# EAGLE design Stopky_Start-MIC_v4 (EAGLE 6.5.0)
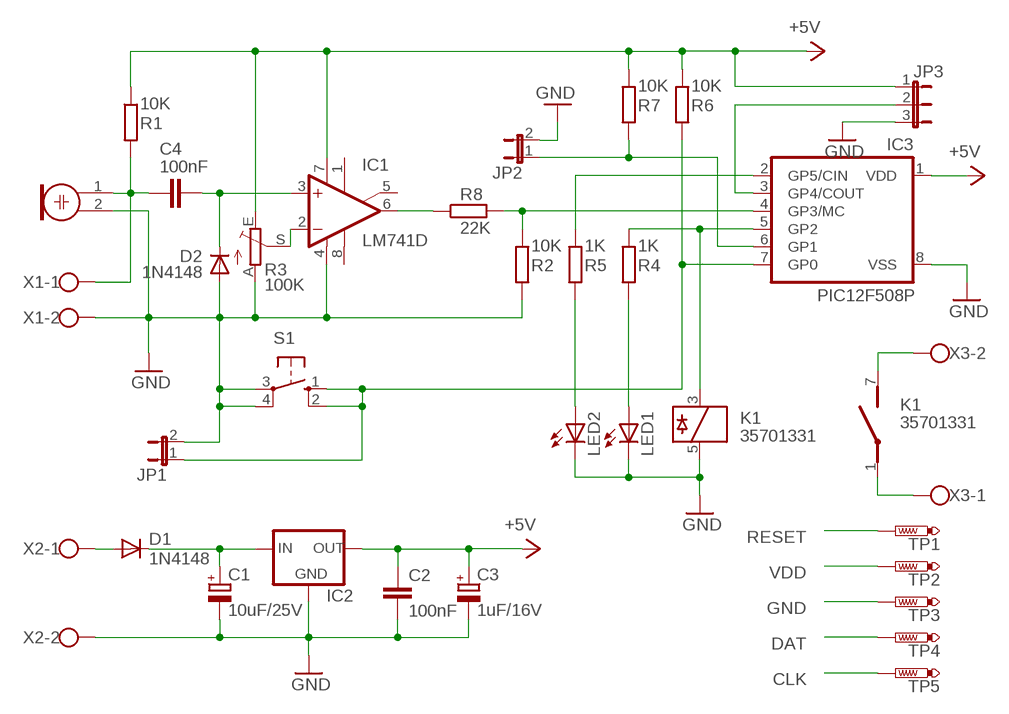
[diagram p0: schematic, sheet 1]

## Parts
C1  10uF/25V  CPOL-EUSMCD  [SMC_D]
C2  100nF  C-EUC1206  [C1206]
C3  1uF/16V  CPOL-EUSMCA  [SMC_A]
C4  100nF  C-EUC1206  [C1206]
D1  1N4148  PMLL4150  [SOD80C]
D2  1N4148  PMLL4150  [SOD80C]
IC1  LM741D  [SO08]
IC2  78LXX-SOT89  [SOT89]
IC3  PIC12F508P  PIC12C508P  [DIL8]
JP1  JP1E  [JP1]
JP2  JP1E  [JP1]
JP3  JP2E  [JP2]
K1  35701331  [REED]
LED1  LED3MM  [LED3MM]
LED2  LED3MM  [LED3MM]
M1  ELECTRET_MIC  ELECTRET_MICROPHON-F6050AP  [F6050AP]
R1  10K  R-EU_R1206  [R1206]
R2  10K  R-EU_R1206  [R1206]
R3  100K  TRIM_EU-CA6V  [CA6V]
R4  1K  R-EU_R1206  [R1206]
R5  1K  R-EU_R1206  [R1206]
R6  10K  R-EU_R1206  [R1206]
R7  10K  R-EU_R1206  [R1206]
R8  22K  R-EU_R1206  [R1206]
S1  10-XX  [B3F-10XX]
TP1  PTR1TP15R  [TP15R]
TP2  PTR1TP15R  [TP15R]
TP3  PTR1TP15R  [TP15R]
TP4  PTR1TP15R  [TP15R]
TP5  PTR1TP15R  [TP15R]
X1  AK550/2  [AK550/2]
X2  AK550/2  [AK550/2]
X3  AK550/2  [AK550/2]

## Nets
+5V: C2.1 C3.+ IC1.7(V+) IC2.1(OUT) IC3.1(VDD) JP3.1 R1.1 R3.E R6.1 R7.1 TP2.TP
GND: C1.- C2.2 C3.- D2.A IC1.4(V-) IC2.2(GND) IC3.8(VSS) JP1.2 JP2.2 JP3.3 K1.5 LED1.K(C) LED2.K(C) M1.2 R2.2 R3.A S1.3(P) S1.4(P1) TP3.TP X1.2 X2.2
GP0: IC3.7(GP0) JP1.1 R6.2 S1.1(S) S1.2(S1) TP4.TP
GP1: IC3.6(GP1) JP2.1 R7.2 TP5.TP
GP3: IC3.4(GP3/MC) R2.1 R8.2 TP1.TP
GP4: IC3.3(GP4/COUT) JP3.2
GP5: IC3.2(GP5/CIN) R5.1
N$1: C4.1 M1.1 R1.2 X1.1
N$2: C4.2 D2.C IC1.3(+IN)
N$3: IC1.2(-IN) R3.S
N$4: K1.7(2:S) X3.2
N$5: IC1.6(OUT) R8.1
N$6: K1.1(2:P) X3.1
N$7: IC3.5(GP2) K1.3 R4.1
N$8: D1.A X2.1
N$9: C1.+ D1.C IC2.3(IN)
N$10: LED1.A R4.2
N$12: LED2.A R5.2
Unconnected: IC1.1(ON1) IC1.5(ON2) IC1.8(OPT)

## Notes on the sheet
- RESET
- VDD
- GND
- DAT
- CLK

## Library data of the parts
C1 C3 = rcl:CPOL-EU: POLARIZED CAPACITOR, European symbol
C2 C4 = rcl:C-EU: CAPACITOR, European symbol
D1 D2 = diode:PMLL4150: DIODE
IC1 = linear:*741: OP AMP
IC2 = v-reg-3:78LXX: VOLTAGE REGULATOR
IC3 = microchip-6:PIC12C*?: MICROCONTROLLER
JP1 JP2 = jumper:JP1E: JUMPER
JP3 = jumper:JP2E: JUMPER
K1 = relay:35701331: RELAY reed, 1 x norm. open with polarity; OC_FARNELL: unknown; OC_NEWARK: unknown
LED1 LED2 = led:LED: LED
M1 = microphon:ELECTRET_MICROPHON-: Electret Condenser Microphone
R1 R2 R4-R8 = rcl:R-EU_: RESISTOR, European symbol
R3 = pot:TRIM_EU-: POTENTIOMETER
S1 = switch-omron:10-XX: OMRON SWITCH; MPN: B3F-1000; OC_FARNELL: 176432; OC_NEWARK: 36M3542
TP1-TP5 = testpad:PTR1: TEST PIN
X1-X3 = con-ptr500+:AK550/2: CONNECTOR

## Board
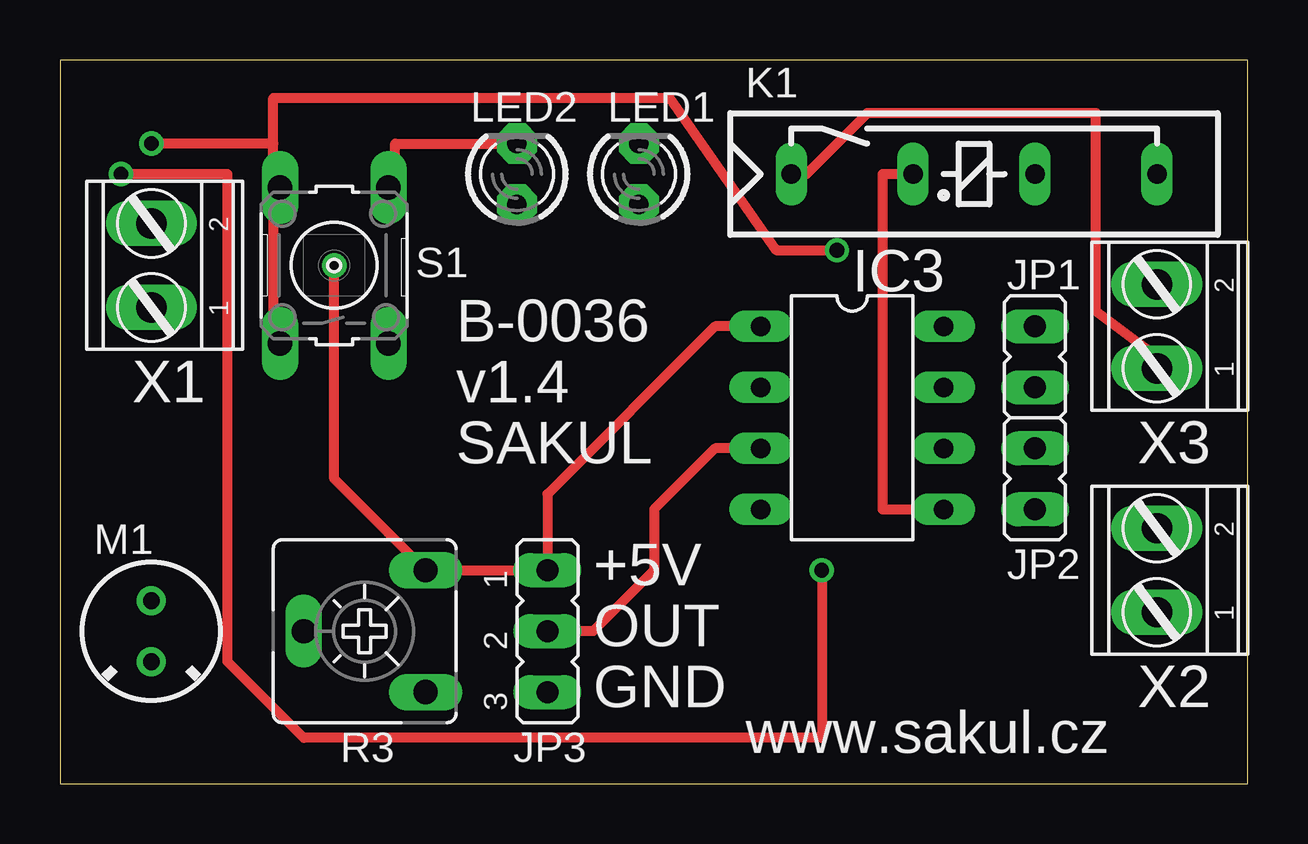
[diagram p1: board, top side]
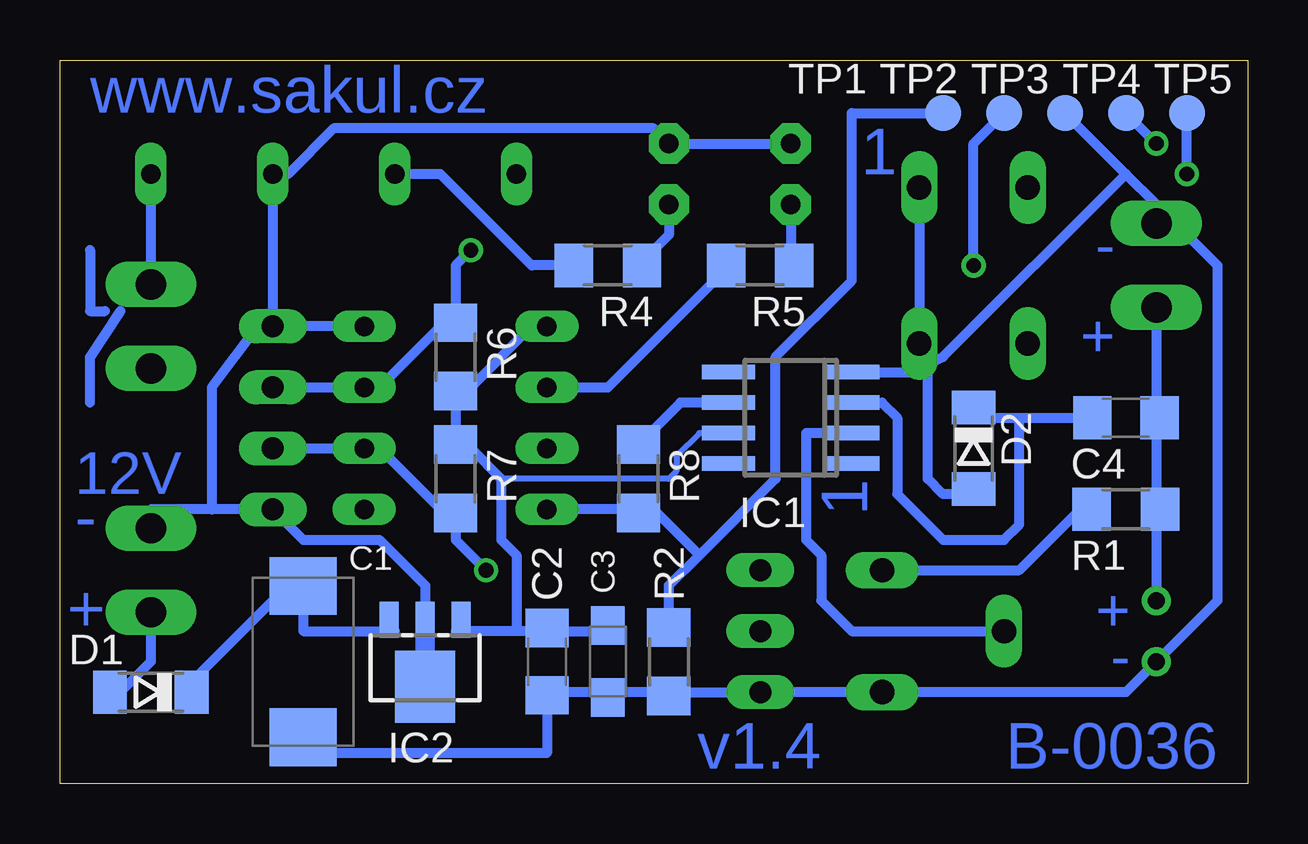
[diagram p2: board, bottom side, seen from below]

Size 49.51 x 30.15 mm. Coordinates in mm from the lower left corner, seen from the top.
Outline: 0,0 49.51,0 49.51,30.15 0,30.15 0,0
Copper layers (1*16): Top 0.035mm / dielectric 1.5mm / Bottom 0.035mm
Design rules "default": minimum track width 10mil, minimum drill 24mil, track to track 8mil, track to pad 8mil, pad to pad 8mil, via to via 8mil, smd to smd 8mil, copper to edge 40mil, drill to drill 8mil, minimum pad ring 10mil, minimum via ring 8mil, stop-mask expansion 4mil, vias tented up to drill 0mil, thermal gap 10mil

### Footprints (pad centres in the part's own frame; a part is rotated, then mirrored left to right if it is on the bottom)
SMC_D = smd 2.4 x 2.8: + -3.15,0; - 3.15,0
C1206 = smd 1.6 x 1.8: 1 -1.4,0; 2 1.4,0
SMC_A = smd 1.6 x 1.4: + -1.5,0; - 1.5,0
SOD80C = smd 1.4 x 1.8: A 1.7,0; C -1.7,0
SO08 = smd 0.6 x 2.2: 1 -1.905,-2.6; 2 -0.635,-2.6; 3 0.635,-2.6; 4 1.905,-2.6; 5 1.905,2.6; 6 0.635,2.6; 7 -0.635,2.6; 8 -1.905,2.6
SOT89 = smd 0.8 x 1.5: 1 -1.5,-1.75; 2 0,-1.75; 3 1.5,-1.75 | smd 2.5 x 3: 4 0,1.05
DIL8 = drill 0.813 long: 1 -3.81,-3.81; 2 -1.27,-3.81; 3 1.27,-3.81; 4 3.81,-3.81; 5 3.81,3.81; 6 1.27,3.81; 7 -1.27,3.81; 8 -3.81,3.81
JP1 = drill 0.914 long: 1 0,-1.27; 2 0,1.27
JP2 = drill 0.914 long: 1 -2.54,0; 2 0,0; 3 2.54,0
REED = drill 0.813 long: 1 -17.78,2.54; 3 -12.7,2.54; 5 -7.62,2.54; 7 -2.54,2.54
LED3MM = drill 0.813 pad 1.676 octagon: A -1.27,0; K 1.27,0
F6050AP = drill 0.7 pad 1.2: 1 0,1.27; 2 0,-1.27
R1206 = smd 1.6 x 1.803: 1 -1.422,0; 2 1.422,0
CA6V = drill 1.016 long: A -2.54,-2.54; E 2.54,-2.54; S 0,2.54
B3F-10XX = drill 1.016 long: 1 -3.251,2.261; 2 3.251,2.261; 3 -3.251,-2.261; 4 3.251,-2.261
TP15R = smd 1.5 x 1.5: TP 0,0
AK550/2 = drill 1.27 long: 1 -1.75,0; 2 1.75,0

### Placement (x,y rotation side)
C1  39.37,5.08 270 bottom
C2  29.21,5.08 270 bottom
C3  26.67,5.08 270 bottom
C4  5.08,15.24 180 bottom
D1  45.72,3.81 180 bottom
D2  11.43,13.97 270 bottom
IC1  19.05,15.24 90 bottom
IC2  34.29,5.08 180 bottom
IC3  33.02,15.24 270 top
JP1  40.64,17.78 0 top
JP2  40.64,12.7 180 top
JP3  20.32,6.35 270 top
K1  48.26,22.86 0 top
LED1  24.13,25.4 90 top
LED2  19.05,25.4 90 top
M1  3.81,6.35 0 top
R1  5.08,11.43 0 bottom
R2  24.13,5.08 270 bottom
R3  12.7,6.35 90 top
R4  26.67,21.59 0 bottom
R5  20.32,21.59 0 bottom
R6  33.02,17.78 90 bottom
R7  33.02,12.7 270 bottom
R8  25.4,12.7 270 bottom
S1  11.43,21.59 90 top
TP1  12.7,27.94 0 bottom
TP2  10.16,27.94 0 bottom
TP3  7.62,27.94 0 bottom
TP4  5.08,27.94 0 bottom
TP5  2.54,27.94 0 bottom
X1  3.81,21.59 90 top
X2  45.72,8.89 90 top
X3  45.72,19.05 90 top

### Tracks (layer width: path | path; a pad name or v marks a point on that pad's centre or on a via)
+5V  (via drill 0.61)
  Top 0.406: v11.43,21.59 11.43,12.7 R3.E JP3.1 20.32,12.06 27.3,19.05 IC3.1
  Bottom 0.254: 33.02,6.35 IC2.1 | 26.67,6.35 C3.+ | 29.21,6.35 C2.1 | 33.02,13.97 R7.1 | 33.02,16.51 R6.1 | 6.99,11.43 R1.1 6.35,11.43 | IC1.7 22.86,14.61 23.81,13.65 23.81,13.02 24.13,12.7 31.11,12.7
  Bottom 0.406: 30.48,6.35 29.21,6.35 26.67,6.35 | 30.48,6.35 33.02,6.35 | R6.1 R7.1 | 30.48,6.35 30.48,9.53 31.11,10.16 31.11,12.7 32.38,13.97 33.02,13.97 | TP2.TP 11.43,26.67 v11.43,21.59 | 6.99,11.43 9.53,8.89 R3.E | 33.02,16.51 32.38,16.51 29.84,19.05 IC3.1
GND
  Top 0.406: LED2.K 13.97,26.67 13.97,25.4 S1.4
  Bottom 0.254: 34.29,6.35 IC2.2 | 26.67,3.81 C3.- | 39.37,1.27 C1.- | 29.21,3.81 C2.2 | 24.13,3.81 R2.2 | 11.43,12.7 D2.A
  Bottom 0.406: IC2.2 34.29,6.99 34.29,8.26 36.2,10.16 39.37,10.16 JP2.2 43.18,11.43 | 29.21,3.81 26.67,3.81 24.13,3.81 JP3.3 R3.A 5.08,3.81 M1.2 1.27,7.62 1.27,21.59 3.81,24.13 | 39.37,1.27 29.21,1.27 C2.2 | 3.81,24.13 5.08,25.4 | 5.08,25.4 TP3.TP | 3.81,24.13 X1.2 | 13.97,17.14 13.21,17.53 | 13.21,17.53 12.7,17.78 5.08,25.4 | IC1.4 13.97,17.14 | 13.97,17.14 13.97,17.78 S1.3 S1.4 | 11.43,12.7 11.43,12.06 12.7,12.06 13.34,12.7 13.34,17.4 13.21,17.53 | 43.18,11.43 45.72,11.43 X2.2 | IC3.8 JP1.2 | JP1.2 41.27,19.05 43.18,16.51 43.18,11.43 | JP1.2 K1.5 40.01,25.4 38.1,27.3 24.77,27.3 LED1.K LED2.K
  Bottom 0.813: 34.29,6.99 34.29,4.45
GP0  (via drill 0.61)
  Top 0.406: 8.89,26.67 v3.81,26.67 | 8.89,26.67 8.89,25.4 S1.2 8.89,24.13 8.89,19.05 S1.1 | v32.38,22.23 29.84,22.23 25.4,28.57 8.89,28.57 8.89,26.67
  Bottom 0.254: 33.02,19.05 R6.2 | 36.2,16.51 IC3.7
  Bottom 0.406: v3.81,26.67 TP4.TP | 33.02,19.05 33.66,19.05 36.2,16.51 | v32.38,22.23 33.02,21.59 R6.2 | JP1.1 IC3.7
GP1  (via drill 0.61)
  Top 0.406: v2.54,25.4 6.99,25.4 6.99,5.08 10.16,1.91 31.75,1.91 v31.75,8.89
  Bottom 0.254: 33.02,11.43 R7.2
  Bottom 0.406: v2.54,25.4 TP5.TP | v31.75,8.89 33.02,10.16 R7.2 | 33.02,11.43 33.66,11.43 36.2,13.97 IC3.6 JP2.1
GP3
  Bottom 0.254: 24.13,6.35 R2.1 | 24.77,11.43 R8.2
  Bottom 0.406: TP1.TP 16.51,27.94 16.51,20.95 19.68,17.78 19.68,12.7 22.86,9.53 | 22.86,9.53 24.13,8.26 R2.1 | 22.86,9.53 24.77,11.43 IC3.4
GP4
  Top 0.406: JP3.2 20.95,6.35 21.59,6.35 22.23,6.35 24.77,8.89 24.77,11.43 27.3,13.97 IC3.3
GP5
  Bottom 0.254: 21.59,21.59 R5.1
  Bottom 0.406: 21.59,21.59 26.67,16.51 IC3.2
N$1
  Bottom 0.254: 3.81,15.24 C4.1 | 3.81,11.43 R1.2
  Bottom 0.406: X1.1 3.81,15.24 3.81,11.43 M1.1
N$2
  Bottom 0.254: 6.35,15.24 C4.2 | 11.43,15.24 D2.C
  Bottom 0.406: 11.43,15.24 9.53,15.24 | 9.53,15.24 C4.2 | IC1.3 15.24,15.88 14.61,15.24 14.61,12.06 12.7,10.16 10.16,10.16 9.53,10.79 9.53,15.24
N$3
  Bottom 0.406: IC1.2 18.41,14.61 18.41,10.16 17.78,9.53 17.78,7.62 16.51,6.35 R3.S
N$4
  Bottom 0.406: K1.7 X3.2
N$5
  Bottom 0.406: IC1.6 23.65,15.88 R8.1
N$6
  Top 0.406: K1.1 31.11,25.4 33.66,27.94 43.18,27.94 43.18,19.68 45.72,17.78 X3.1
N$7
  Top 0.406: IC3.5 34.29,11.43 34.29,25.4 K1.3
  Bottom 0.254: 27.94,21.59 R4.1
  Bottom 0.406: R4.1 29.84,21.59 33.66,25.4 K1.3
N$8
  Bottom 0.254: 46.99,3.81 D1.A
  Bottom 0.406: 46.99,3.81 45.72,5.08 X2.1
N$9
  Bottom 0.254: 35.56,6.35 IC2.3 | 44.45,3.81 D1.C | 39.37,8.89 C1.+
  Bottom 0.406: 35.56,6.35 39.37,6.35 C1.+ | 39.37,8.89 44.45,3.81
N$10
  Bottom 0.254: 25.4,21.59 R4.2
  Bottom 0.406: 25.4,21.59 24.13,22.86 LED1.A
N$11
  Bottom 0.406: 48.26,15.88 48.26,17.78 46.99,19.68
N$12
  Bottom 0.254: 19.05,21.59 R5.2
  Bottom 0.406: LED2.A 19.05,21.59
N$13
  Bottom 0.406: 48.26,22.23 48.26,19.68 47.62,19.68

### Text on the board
Bottom: www.sakul.cz | 1 | - | + | 1 | 12V | - | + | + | - | B-0036 | v1.4
tPlace: B-0036 | v1.4 | SAKUL | +5V | OUT | GND | www.sakul.cz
